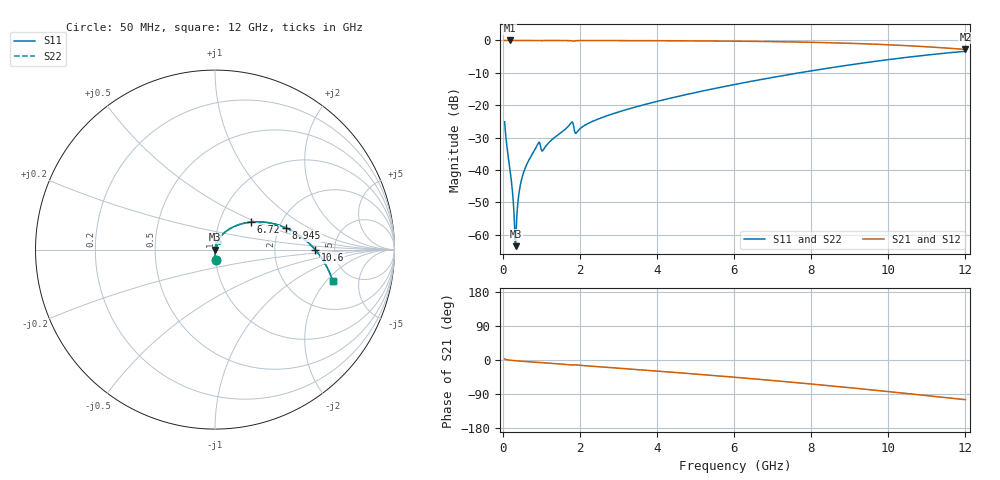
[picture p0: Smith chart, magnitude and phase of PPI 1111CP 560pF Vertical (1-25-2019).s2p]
# GHz S MA R 50
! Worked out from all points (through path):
!   1601 points, 50 MHz to 12 GHz, reference 50 ohm
!   highest |S21| = 0.00 dB at 184.4 MHz (marker M1); lowest = -2.8 dB at 12 GHz (marker M2)
!   group delay of S21, straight-line fit = 24.1 ps
!   lowest |S11| = -63.5 dB at 333.8 MHz (marker M3), VSWR 1.00, Z = 50.1 + j0.0159 ohm
!   |S11| at or under -10 dB: start of sweep to 7.692 GHz
!   |S22| runs from -63.5 to -3.3 dB; largest |S21 - S12| = 0
!   S11 on the Smith chart (normalised r, x): 50 MHz: 1.00, -0.11; 6.72 GHz: 1.41, +0.46; 8.945 GHz: 2.19, +0.64; 10.6 GHz: 3.53, -0.01; 12 GHz: 3.60, -2.38
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0.05  0.05541 -86.8  0.9982 2.9  0.9982 2.9  0.05541 -86.8
0.1844375  0.01063 -87.7  0.9994 -0.5  0.9994 -0.5  0.01063 -87.7
0.2367188  0.005882 -85.6  0.9994 -1.0  0.9994 -1.0  0.005882 -85.6
0.289  0.002395 -77.0  0.9994 -1.5  0.9994 -1.5  0.002395 -77.0
0.3338125  0.0006652 13.8  0.9993 -1.9  0.9993 -1.9  0.0006652 13.8
0.3711563  0.002133 69.4  0.9993 -2.3  0.9993 -2.3  0.002133 69.4
0.4458437  0.005357 79.3  0.9992 -2.9  0.9992 -2.9  0.005357 79.3
0.5205313  0.0083 81.1  0.9991 -3.5  0.9991 -3.5  0.0083 81.1
0.8939687  0.02395 76.1  0.9966 -6.5  0.9966 -6.5  0.02395 76.1
1.058281  0.02063 72.3  0.996 -7.2  0.996 -7.2  0.02063 72.3
1.767813  0.05286 67.8  0.9902 -13.1  0.9902 -13.1  0.05286 67.8
1.909719  0.0373 63.9  0.9908 -13.0  0.9908 -13.0  0.0373 63.9
2.044156  0.04526 72.0  0.9959 -14.3  0.9959 -14.3  0.04526 72.0
2.723813  0.06927 68.9  0.9956 -19.5  0.9956 -19.5  0.06927 68.9
4.038312  0.1159 59.4  0.9908 -29.5  0.9908 -29.5  0.1159 59.4
6.025  0.2093 43.6  0.9747 -45.6  0.9747 -45.6  0.2093 43.6
6.719594  0.2504 37.7  0.9647 -51.6  0.9647 -51.6  0.2504 37.7
8.019156  0.3405 25.9  0.9362 -63.5  0.9362 -63.5  0.3405 25.9
8.945281  0.4143 16.9  0.9056 -72.6  0.9056 -72.6  0.4143 16.9
10.01331  0.5066 6.0  0.857 -83.5  0.857 -83.5  0.5066 6.0
10.59587  0.5585 -0.1  0.824 -89.6  0.824 -89.6  0.5585 -0.1
12  0.6805 -15.1  0.7265 -104.6  0.7265 -104.6  0.6805 -15.1
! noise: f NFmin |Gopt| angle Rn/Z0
0.05  0.0003804  0.8688  0.3193  0.0006238
1.372  0.00458  0.725  7.781  0.003293
2.701  0.006971  0.6615  15.08  0.003874
4.031  0.009147  0.6297  22.09  0.004474
5.36  0.01145  0.6193  28.81  0.00528
6.682  0.01384  0.62  35.19  0.006207
8.012  0.01643  0.629  41.28  0.007328
9.341  0.0193  0.6449  47.08  0.008728
10.67  0.02258  0.6663  52.62  0.01054
12  0.02643  0.6924  57.94  0.01294
